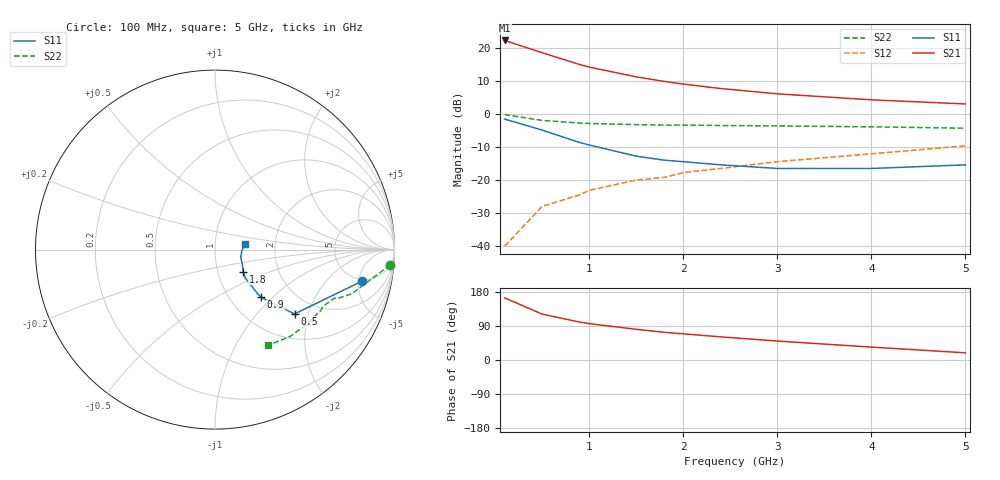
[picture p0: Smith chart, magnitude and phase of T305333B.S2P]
!AT-30533
!S and NOISE PARAMETERS at Vce=2.7V  Ic=5mA.  LAST UPDATED 04-10-94
# ghz s ma r 50!
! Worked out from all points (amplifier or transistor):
!   11 points, 100 MHz to 5 GHz, reference 50 ohm
!   highest |S21| = 22.3 dB at 100 MHz (marker M1)
!   |S21| within 3 dB of that: start of sweep to 422.7 MHz
!   unconditionally stable (mu >= 1): 1.566 GHz to 3.271 GHz
!   at 500 MHz: K = 0.69, MSG = 23.3 dB, |S12| = -28.0 dB
!   at 1.8 GHz: K = 1.05, MAG = 13.2 dB, |S12| = -19.2 dB
!   at 5 GHz: K = 0.93, MSG = 6.3 dB, |S12| = -9.6 dB
!   lowest NFmin = 1.10 dB at 500 MHz
!   S11 on the Smith chart (normalised r, x): 100 MHz: 4.72, -5.61; 500 MHz: 1.54, -1.63; 900 MHz: 1.39, -0.85; 1.8 GHz: 1.32, -0.34; 5 GHz: 1.40, +0.09
0.1  0.84 -12.0  12.98 164.0  0.01 82.0  0.98 -5.0
0.5  0.57 -39.0  8.46 121.0  0.04 71.0  0.8 -18.0
0.9  0.37 -46.0  5.6 100.0  0.06 70.0  0.73 -22.0
1  0.34 -46.0  5.13 96.0  0.07 69.0  0.72 -22.0
1.5  0.23 -43.0  3.65 81.0  0.1 68.0  0.69 -26.0
1.8  0.2 -38.0  3.11 73.0  0.11 67.0  0.68 -28.0
2  0.19 -35.0  2.84 69.0  0.13 66.0  0.68 -30.0
2.4  0.17 -27.0  2.43 61.0  0.15 64.0  0.67 -33.0
3  0.15 -17.0  2.02 50.0  0.19 61.0  0.66 -39.0
4  0.15 -2.0  1.64 34.0  0.25 55.0  0.64 -49.0
5  0.17 11.0  1.42 19.0  0.33 47.0  0.61 -61.0
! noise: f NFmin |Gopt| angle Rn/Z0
0.5  1.1  0.71  8  0.78
0.9  1.2  0.61  16  0.66
1.8  1.5  0.42  39  0.41
2.4  1.8  0.28  57  0.25
